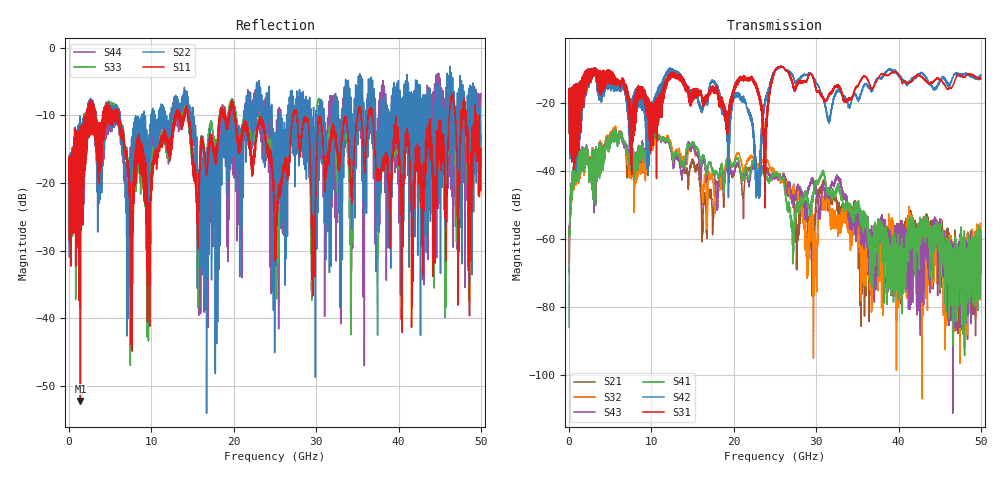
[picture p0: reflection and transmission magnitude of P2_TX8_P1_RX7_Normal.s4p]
!Keysight Technologies,N5225B,MY57041031,A.13.20.10
!Date: Friday, May 31, 2019 11:25:28
!Correction: S11(Full 4 Port(1,2,3,4))
!S12(Full 4 Port(1,2,3,4))
!S13(Full 4 Port(1,2,3,4))
!S14(Full 4 Port(1,2,3,4))
!S21(Full 4 Port(1,2,3,4))
!S22(Full 4 Port(1,2,3,4))
!S23(Full 4 Port(1,2,3,4))
!S24(Full 4 Port(1,2,3,4))
!S31(Full 4 Port(1,2,3,4))
!S32(Full 4 Port(1,2,3,4))
!S33(Full 4 Port(1,2,3,4))
!S34(Full 4 Port(1,2,3,4))
!S41(Full 4 Port(1,2,3,4))
!S42(Full 4 Port(1,2,3,4))
!S43(Full 4 Port(1,2,3,4))
!S44(Full 4 Port(1,2,3,4))
!S4P File: Measurements: <S11,S12,S13,S14>,
!<S21,S22,S23,S24>,
!<S31,S32,S33,S34>,
!<S41,S42,S43,S44>:
# Hz S  dB  R 50.0
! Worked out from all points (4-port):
!   5000 points, 10 MHz to 50 GHz, reference 50 ohm
!   strongest paths, dB at 10 MHz, 12.51 GHz, 25.01 GHz, 37.51 GHz, 50 GHz:
!     S31: -19.4, -11.5, -10.3, -12.8, -12.8
!     S42: -19.6, -10.0, -10.6, -12.5, -11.8
!     S41: -86.0, -35.1, -41.2, -54.1, -57.3
!     S43: -69.1, -36.3, -41.9, -57.0, -63.9
!     S32: -67.0, -33.3, -41.1, -58.1, -69.0
!     S21: -56.8, -35.1, -40.7, -62.2, -69.7
!   lowest |S11| = -52.2 dB at 1.38 GHz (marker M1), VSWR 1.00, Z = 49.9 - j0.206 ohm
!   |S11| at or under -10 dB: 20.17 GHz to 27.18 GHz (7.011 GHz wide, 29.6 % of centre); 27.67 GHz to 35.04 GHz (7.369 GHz wide, 23.5 % of centre); 36.79 GHz to 46.16 GHz (9.374 GHz wide, 22.6 % of centre)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
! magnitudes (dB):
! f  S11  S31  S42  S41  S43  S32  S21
! 10 MHz  -19.5  -19.4  -19.6  -86.0  -69.1  -67.0  -56.8
! 1.38 GHz  -52.2  -28.8  -23.6  -36.7  -36.2  -37.1  -37.1
! 17.51 GHz  -14.5  -15.8  -13.4  -40.1  -39.7  -43.0  -53.3
! 22.93 GHz  -11.7  -16.6  -40.1  -42.7  -41.6  -38.9  -42.1
! 25.47 GHz  -21.2  -9.4  -9.4  -41.2  -41.0  -41.2  -41.3
! 29.91 GHz  -22.6  -15.3  -13.3  -43.7  -46.2  -62.5  -54.1
! 50 GHz  -15.0  -12.8  -11.8  -57.3  -63.9  -69.0  -69.7
